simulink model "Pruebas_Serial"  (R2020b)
settings: Solver=VariableStepAuto  StartTime=0.0  StopTime=inf  RelTol=1e-3
undefined symbols (not defined in the file or in its folder): serial
libraries: instrumentlib x4

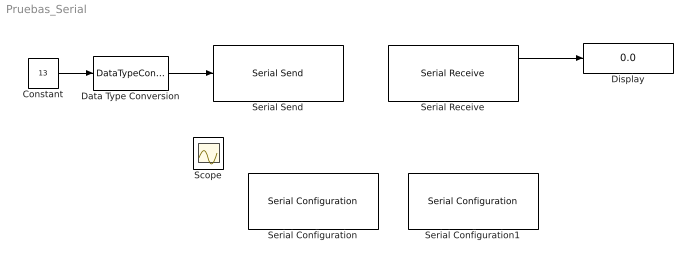
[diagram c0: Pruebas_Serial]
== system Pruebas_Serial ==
  Constant : Constant  Value=13  OutDataTypeStr=single  SampleTime=0.1
  Data Type Conversion : DataTypeConversion  OutDataTypeStr=single
  Display : Display
  Scope : Scope
  Serial Configuration : instrumentlib/Serial Configuration  Priority=-200000  ComPortMenu=COM1  ComPort=COM1  ObjConstructor=serial('COM1');  BaudRate=9600  DataBits=8  Parity=none  StopBits=1  FlowControl=none  Timeout=10  ByteOrder=LittleEndian
  Serial Configuration1 : instrumentlib/Serial Configuration  Priority=-200000  Commented=on  ComPortMenu=COM2  ComPort=COM2  ObjConstructor=serial('COM2');  BaudRate=9600  DataBits=8  Parity=none  StopBits=1  FlowControl=none  Timeout=10  ByteOrder=LittleEndian
  Serial Receive : instrumentlib/Serial Receive  Commented=on  ComPortMenu=COM2  ComPort=COM2  ObjConstructor=serial('COM2');  Terminator=<none>  DataSize=[1 1]  DataType=single  EnableBlockingMode=off  ActionDataUnavailable=Output last received value  CustomValue=0  SampleTime=0.01
  Serial Send : instrumentlib/Serial Send  ComPortMenu=COM1  ComPort=COM1  ObjConstructor=serial('COM1');  Terminator=<none>  EnableBlockingMode=off
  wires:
  Serial Receive/1 -> Display/1
  Constant/1 -> Data Type Conversion/1
  Data Type Conversion/1 -> Serial Send/1
